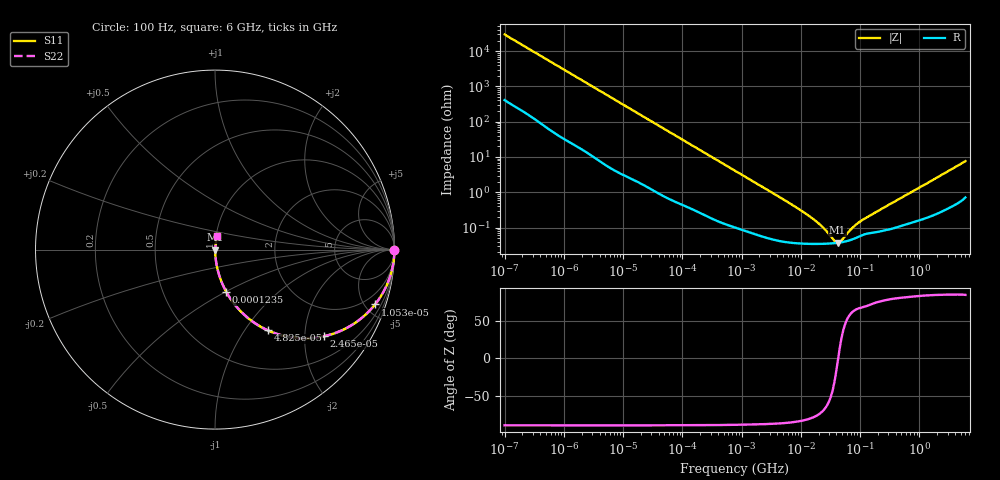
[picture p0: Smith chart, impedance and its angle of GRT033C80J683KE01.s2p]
!Murata Part Number: GRT033C80J683KE01
!These Parameters are Measured in Series Mode Connection
!Data Generated on Jun 19, 2026
!  o--ll--o
!Port1  Port2
!  o------o
!Operation Temp=25[degC], DC Bias Voltage=0[V]
!Freq. Start=100[Hz] Stop=6[GHz] 401[Steps]
# Hz S RI R 50
!Freq.(Hz) S11(Real) S11(Imag) S21(Real) S21(Imag) S12(Real) S12(Imag) S22(Real) S22(Imag)
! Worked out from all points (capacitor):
!   401 points, 100 Hz to 6 GHz, reference 50 ohm
!   read as one part in series: C = 53.5 nF near 109 Hz
!   lowest |Z| = 37.3 mohm at 41.66 MHz (marker M1)
!   series resonance near 42.75 MHz, so ESL is about 260 pH
!   S11 on the Smith chart (normalised r, x): 100 Hz: open; 10.53 kHz: 1.06, -5.82; 24.65 kHz: 1.03, -2.50; 48.25 kHz: 1.02, -1.28; 123.5 kHz: 1.01, -0.50; 6 GHz: 1.01, +0.15
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100  0.9999 -0.00337  5.8e-05 0.00337  5.8e-05 0.00337  0.9999 -0.00337
2008  0.9949 -0.0658  0.00507 0.0658  0.00507 0.0658  0.9949 -0.0658
4918  0.9732 -0.1565  0.0268 0.1565  0.0268 0.1565  0.9732 -0.1565
10527  0.8919 -0.3054  0.1081 0.3054  0.1081 0.3054  0.8919 -0.3054
15752  0.7892 -0.4023  0.2108 0.4023  0.2108 0.4023  0.7892 -0.4023
24648  0.6088 -0.4822  0.3912 0.4822  0.3912 0.4822  0.6088 -0.4822
40335  0.3719 -0.4774  0.6281 0.4774  0.6281 0.4774  0.3719 -0.4774
48246  0.2942 -0.4496  0.7058 0.4496  0.7058 0.4496  0.2942 -0.4496
75495  0.1481 -0.3487  0.8519 0.3487  0.8519 0.3487  0.1481 -0.3487
123542  0.063 -0.2357  0.937 0.2357  0.937 0.2357  0.063 -0.2357
276587  0.0147 -0.1118  0.9853 0.1118  0.9853 0.1118  0.0147 -0.1118
774597  0.00268 -0.0408  0.9973 0.0408  0.9973 0.0408  0.00268 -0.0408
6075234  0.000409 -0.00524  0.9996 0.00524  0.9996 0.00524  0.000409 -0.00524
1.555665e7  0.000349 -0.00181  0.9997 0.00181  0.9997 0.00181  0.000349 -0.00181
2.434276e7  0.000349 -0.000903  0.9997 0.000903  0.9997 0.000903  0.000349 -0.000903
3.64232e7  0.000363 -0.000244  0.9996 0.000244  0.9996 0.000244  0.000363 -0.000244
4.165952e7  0.000371 -3.88e-05  0.9996 3.88e-05  0.9996 3.88e-05  0.000371 -3.88e-05
4.764863e7  0.000383 0.000165  0.9996 -0.000165  0.9996 -0.000165  0.000383 0.000165
7.129496e7  0.000454 0.0008  0.9995 -0.0008  0.9995 -0.0008  0.000454 0.0008
9.753859e7  0.000568 0.00133  0.9994 -0.00133  0.9994 -0.00133  0.000568 0.00133
3.124326e8  0.000911 0.00444  0.9991 -0.00444  0.9991 -0.00444  0.000911 0.00444
6e9  0.0128 0.0748  0.9872 -0.0748  0.9872 -0.0748  0.0128 0.0748
